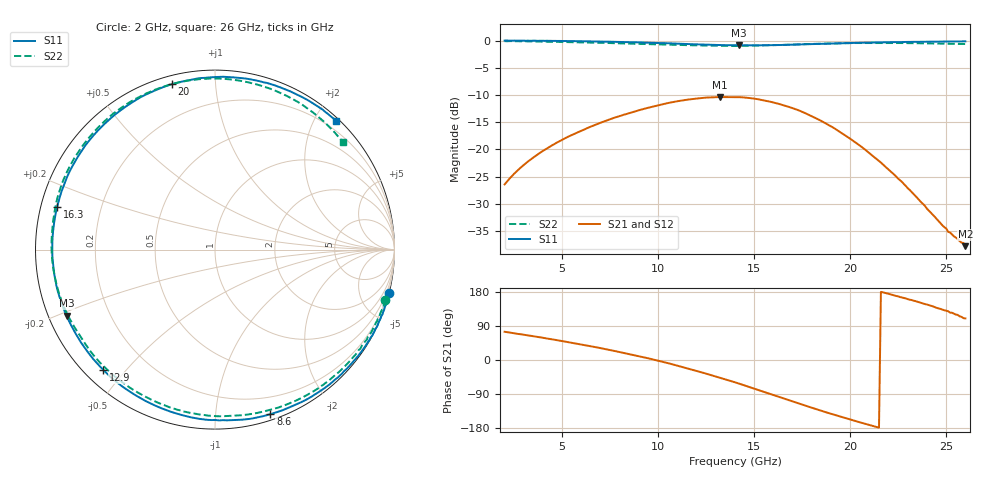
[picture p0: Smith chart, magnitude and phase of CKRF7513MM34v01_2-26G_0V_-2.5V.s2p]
! CHUO DENSHI KOGYO Co.,Ltd.
! 1. March 2016
! CKRF7513MM34
! N-channel HJ-FET
! Vds = 0 V Vgs = -2.5 V
# Hz S  MA  R 50
!  f  S11  S21  S12  S22
!  Hz  MAG  ANG  MAG  ANG  MAG  ANG  MAG  ANG
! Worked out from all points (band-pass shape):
!   241 points, 2 GHz to 26 GHz, reference 50 ohm
!   highest |S21| = -10.37 dB at 13.2 GHz (marker M1); lowest = -37.8 dB at 26 GHz (marker M2)
!   |S21| within 3 dB of the highest: 8.458 GHz to 17.68 GHz (9.223 GHz wide, 70.6 % of centre)
!   lowest |S11| = -0.9 dB at 14.2 GHz (marker M3), VSWR 20.11, Z = 2.6 - j10.6 ohm
!   |S11| at or under -10 dB: nowhere
!   |S22| runs from -1.0 to -0.1 dB; largest |S21 - S12| = 0.0012
!   S11 on the Smith chart (normalised r, x): 2 GHz: -0.05, -8.21; 8.6 GHz: 0.05, -1.39; 12.9 GHz: 0.05, -0.44; 16.3 GHz: 0.05, +0.13; 20 GHz: 0.04, +0.77; 26 GHz: 0.05, +2.32
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2e9  1.001 -13.9  0.0477 74.5  0.04759 74.2  0.99 -16.4
3.5e9  0.9994 -24.9  0.08457 62.6  0.08434 62.6  0.9818 -28.9
6e9  0.988 -45.2  0.1484 40.9  0.1486 41.0  0.9649 -51.3
8.6e9  0.9677 -71.4  0.2185 14.5  0.2183 14.6  0.9378 -77.7
1e10  0.952 -88.6  0.2546 -1.8  0.2546 -1.8  0.9236 -93.6
1.14e10  0.9331 -108.5  0.2846 -20.3  0.2845 -20.2  0.9096 -111.0
1.29e10  0.9145 -132.8  0.3018 -42.1  0.3018 -42.0  0.8994 -131.2
1.32e10  0.912 -138.1  0.3031 -46.6  0.3027 -46.5  0.8984 -135.4
1.4e10  0.9057 -152.4  0.3024 -58.8  0.3027 -58.7  0.8923 -146.9
1.42e10  0.9053 -156.0  0.3024 -62.1  0.3025 -62.0  0.8935 -149.7
1.53e10  0.9066 -176.6  0.2869 -80.7  0.2871 -80.5  0.9034 -166.4
1.63e10  0.9113 164.7  0.2617 -97.5  0.261 -97.3  0.9114 177.7
1.72e10  0.9208 148.5  0.2328 -112.6  0.2324 -112.4  0.9224 163.3
1.8e10  0.9302 134.8  0.202 -126.0  0.2021 -125.8  0.9327 150.3
1.9e10  0.9417 119.0  0.1629 -142.0  0.1626 -141.9  0.9417 134.1
2e10  0.9524 104.7  0.1255 -157.2  0.1254 -156.9  0.9493 118.3
2.1e10  0.9598 92.1  0.09236 -171.6  0.09257 -171.4  0.9529 103.1
2.2e10  0.9674 80.8  0.06527 174.8  0.06506 174.7  0.9531 88.7
2.3e10  0.9731 70.9  0.04396 160.5  0.044 161.1  0.9489 75.1
2.41e10  0.9783 61.2  0.02733 144.7  0.02736 145.1  0.9435 61.3
2.56e10  0.9832 49.5  0.01497 119.0  0.01442 118.9  0.9332 44.4
2.6e10  0.9851 46.7  0.0129 109.8  0.01332 110.7  0.9311 40.2
